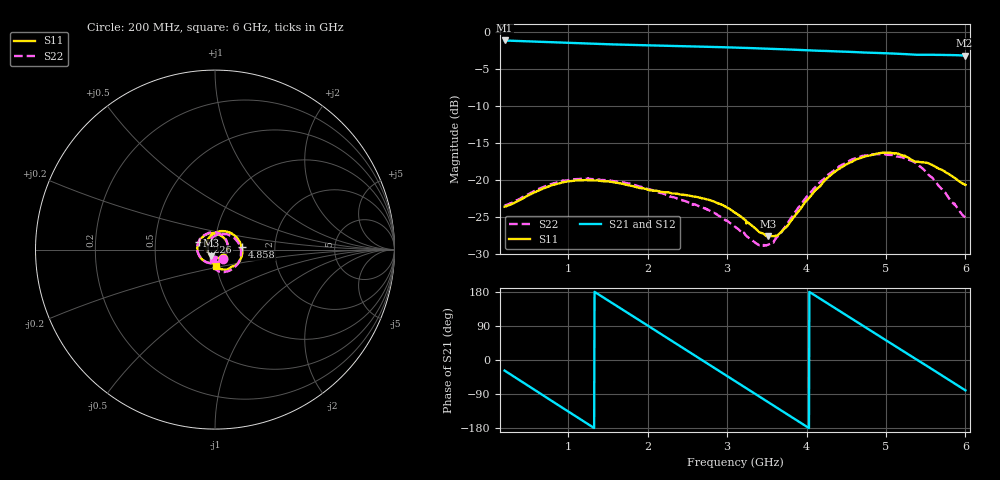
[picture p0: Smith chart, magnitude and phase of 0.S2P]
!Agilent Technologies,E5071C,MY46316741,A.11.02
!Date: Fri Apr 15 16:18:20 2022
!Data & Calibration Information:
!Freq	S11:SOLT2(ON)	S21:SOLT2(ON)	S12:SOLT2(ON)	S22:SOLT2(ON)
!PortZ  Port1:50+j0  Port2:50+j0
!Above PortZ is port z conversion or system Z0 setting when saving the data.
!When reading, reference impedance value at option line is always used.
# Hz S dB R 50
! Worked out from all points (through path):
!   1200 points, 200 MHz to 6 GHz, reference 50 ohm
!   highest |S21| = -1.12 dB at 200 MHz (marker M1); lowest = -3.2 dB at 5.99 GHz (marker M2)
!   group delay of S21, straight-line fit = 370 ps
!   lowest |S11| = -27.6 dB at 3.518 GHz (marker M3), VSWR 1.09, Z = 47.6 - j3.25 ohm
!   |S11| at or under -10 dB: start of sweep to end of sweep
!   |S22| runs from -29.0 to -16.5 dB; largest |S21 - S12| = 0.0026
!   S11 on the Smith chart (normalised r, x): 200 MHz: 1.09, -0.11; 1.226 GHz: 0.83, +0.08; 4.858 GHz: 1.35, +0.04; 6 GHz: 1.00, -0.19
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2e8  -23.61 -47.9  -1.12 -27.9  -1.12 -27.9  -23.45 -49.5
4.563803e8  -22.33 -96.7  -1.23 -62.6  -1.23 -62.6  -22.14 -100.8
6.740617e8  -21.21 -132.5  -1.32 -92.0  -1.32 -92.0  -21.03 -138.6
9.014178e8  -20.41 -165.5  -1.40 -122.6  -1.40 -122.5  -20.22 -173.5
1.167473e9  -20.05 160.3  -1.51 -158.2  -1.51 -158.2  -19.84 150.2
1.225521e9  -20.02 153.3  -1.53 -166.0  -1.53 -165.9  -19.85 142.7
1.472227e9  -20.19 126.2  -1.62 161.1  -1.62 161.2  -20.02 113.0
1.743119e9  -20.67 99.2  -1.71 125.2  -1.71 125.2  -20.44 82.8
2.134946e9  -21.51 65.8  -1.81 73.1  -1.81 73.1  -21.68 42.9
2.401001e9  -21.94 42.6  -1.87 37.6  -1.87 37.6  -22.65 17.9
2.628357e9  -22.32 20.8  -1.94 7.3  -1.94 7.3  -23.47 -4.3
2.855713e9  -23.02 -4.5  -2.01 -23.0  -2.01 -23.0  -24.54 -30.2
3.102419e9  -24.44 -38.1  -2.09 -56.0  -2.09 -55.9  -26.32 -65.6
3.518432e9  -27.65 -124.7  -2.24 -111.4  -2.24 -111.3  -28.76 -162.7
3.808674e9  -25.50 157.8  -2.36 -150.1  -2.35 -150.0  -25.13 124.8
4.069892e9  -21.94 107.1  -2.48 175.2  -2.47 175.3  -21.45 79.9
4.49558e9  -17.93 47.3  -2.65 118.8  -2.64 118.8  -17.70 22.9
4.858382e9  -16.51 5.0  -2.81 70.8  -2.81 70.9  -16.51 -20.0
5.037364e9  -16.30 -14.7  -2.87 47.2  -2.87 47.2  -16.60 -39.7
5.496914e9  -17.64 -54.6  -3.06 -13.2  -3.06 -13.1  -18.83 -85.3
5.990325e9  -20.60 -84.8  -3.16 -78.8  -3.17 -78.8  -25.01 -101.7
6e9  -20.66 -85.0  -3.16 -80.1  -3.17 -80.0  -25.13 -101.3
